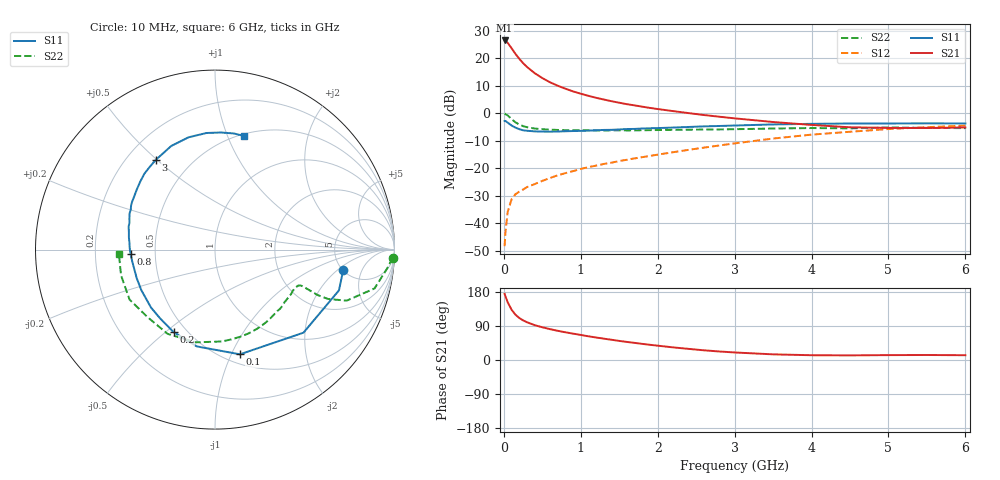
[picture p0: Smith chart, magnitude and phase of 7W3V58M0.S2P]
! Infineon Technologies  Discrete & RF Semiconductors
! BFS17W
! Si NPN RF Bipolar Junction Transistor in SOT323
! VCE = 3.5 V  IC = 8 mA
! Common Emitter S-Parameters:  August  1999
# GHz  S  MA  R  50
!  f  S11  S21  S12  S22
! GHz  MAG  ANG  MAG  ANG  MAG  ANG  MAG  ANG
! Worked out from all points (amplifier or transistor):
!   36 points, 10 MHz to 6 GHz, reference 50 ohm
!   highest |S21| = 26.5 dB at 10 MHz (marker M1)
!   |S21| within 3 dB of that: start of sweep to 104.5 MHz
!   unconditionally stable (mu >= 1): 440 MHz to 2.549 GHz; 4.453 GHz to end of sweep
!   at 250 MHz: K = 0.74, MSG = 23.0 dB, |S12| = -27.8 dB
!   at 1.4 GHz: K = 1.22, MAG = 8.3 dB, |S12| = -18.0 dB
!   at 6 GHz: K = 1.07, MAG = -1.9 dB, |S12| = -4.5 dB
!   S11 on the Smith chart (normalised r, x): 10 MHz: 5.06, -2.40; 100 MHz: 0.59, -1.08; 200 MHz: 0.43, -0.53; 800 MHz: 0.36, -0.02; 3 GHz: 0.32, +0.50; 6 GHz: 0.52, +1.15
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0.01  0.7235 -9.0  21.22 174.6  0.0038 84.4  0.9905 -2.6
0.02  0.727 -18.2  21.06 168.3  0.0066 83.8  0.967 -6.0
0.05  0.6762 -43.2  19.23 152.4  0.016 71.8  0.9148 -13.7
0.1  0.5997 -76.6  15.34 132.9  0.027 59.2  0.7866 -21.2
0.15  0.5489 -100.6  12.15 119.7  0.0335 53.9  0.6868 -23.6
0.2  0.5143 -116.7  9.868 111.0  0.0373 52.7  0.6251 -23.9
0.25  0.4901 -128.7  8.208 104.6  0.0408 51.3  0.5835 -23.4
0.3  0.481 -137.8  7.005 99.7  0.0452 52.7  0.5589 -23.1
0.4  0.4686 -151.2  5.395 92.0  0.0513 54.3  0.5278 -22.7
0.5  0.4643 -160.0  4.379 86.4  0.0587 57.4  0.5131 -22.8
0.6  0.4628 -166.8  3.672 81.4  0.0662 59.6  0.5036 -23.6
0.7  0.466 -172.2  3.181 77.1  0.0743 60.9  0.4974 -24.9
0.8  0.471 -177.1  2.806 73.1  0.0813 61.9  0.4928 -26.6
1.1  0.4849 171.7  2.079 62.5  0.1045 64.3  0.4886 -32.5
1.3  0.4979 165.1  1.78 56.3  0.1196 65.3  0.486 -37.3
1.6  0.517 157.0  1.465 47.7  0.1425 66.4  0.4876 -44.7
2.2  0.5497 142.4  1.096 33.3  0.1954 67.5  0.4993 -61.7
3  0.599 123.4  0.809 19.9  0.283 65.0  0.5132 -85.8
3.5  0.6267 112.9  0.694 14.9  0.3466 61.1  0.5281 -101.9
4.5  0.6514 94.2  0.556 12.2  0.4607 48.9  0.532 -135.3
5.5  0.6556 80.8  0.539 13.2  0.5584 36.2  0.5427 -164.6
6  0.6533 75.5  0.553 12.6  0.5967 30.1  0.5362 -177.4
